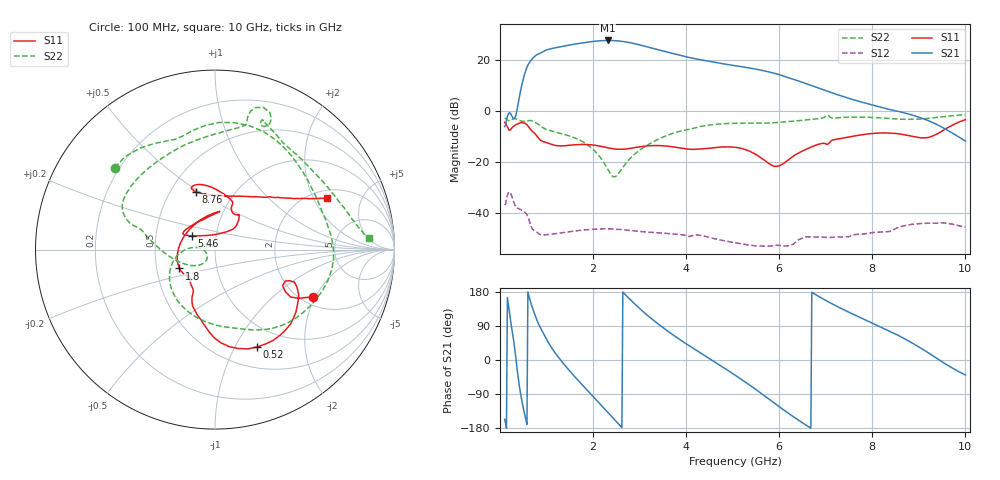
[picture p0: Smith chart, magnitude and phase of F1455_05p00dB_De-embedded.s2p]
! Integrated Device Technology
! Corporate Headquarters
! 6024 Silver Creek Valley Road
! San Jose, CA 95138  USA
! Phone:  1-408-284-8200
! Toll Free:  1-800-223-1366
! Webpage:  http://www.idt.com/
! Timing and RF Division
! 515 Groton Road, Suite 102
! Westford, MA 01886-6024
! Device:  F1455
! Description: 6-bit 0.5 dB Transmit Variable Gain Amplifier
! Frequency:  1400.0 -  2300.00 MHz
! Package:  6x6 mm Thin QFN Plastic Package: 28 pin
! State:  10
! Atten State:  5.0 dB
! Voltage:  +5.00 Volts
! Current:  216.802 mA
! Data:  The device was measured on a the F1455 evaluation board which has
!  individual transmission lines to the RF pins.  Data was collected
!  using a calibrated network analyzer.  The evaluation board was
!  de-embedded using a TRL calibration technique.
!  The reference plane is the edge of the package pin.
!  Pin  1 = CSb
!  Pin  2 = DATA
!  Pin  3 = CLK
!  Pin  4 = RSET
!  Pin  5 = GND
!  Pin  6 = RFIN  = Port 1
!  Pin  7 = GND
!  Pin  8 = NC
!  Pin  9 = NC
!  Pin 10 = NC
!  Pin 11 = NC
!  Pin 12 = NC
!  Pin 13 = NC
!  Pin 14 = /STBY
!  Pin 15 = GND
!  Pin 16 = RFOUT  = Port 2
!  Pin 17 = GND
!  Pin 18 = NC
!  Pin 19 = NC
!  Pin 20 = NC
!  Pin 21 = GND
!  Pin 22 = NC
!  Pin 23 = GND
!  Pin 24 = NC
!  Pin 25 = NC
!  Pin 26 = NC
!  Pin 27 = GND
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# GHz S dB R 50
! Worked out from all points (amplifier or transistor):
!   496 points, 100 MHz to 10 GHz, reference 50 ohm
!   highest |S21| = 27.8 dB at 2.32 GHz (marker M1)
!   |S21| within 3 dB of that: 1.159 GHz to 3.266 GHz (2.107 GHz wide, 95.3 % of centre)
!   unconditionally stable (mu >= 1): start of sweep to end of sweep
!   at 1.74 GHz: K = 4.40, MAG = 27.3 dB, |S12| = -46.7 dB
!   at 5.06 GHz: K = 15.28, MAG = 19.9 dB, |S12| = -51.6 dB
!   at 10 GHz: K = 48.04, MAG = -3.0 dB, |S12| = -45.4 dB
!   S11 on the Smith chart (normalised r, x): 100 MHz: 2.29, -1.92; 520 MHz: 0.74, -1.23; 1.8 GHz: 0.66, -0.15; 5.46 GHz: 0.76, +0.12; 8.76 GHz: 0.67, +0.48; 10 GHz: 2.34, +2.55
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0.1  -4.33 -25.8  -5.96 -156.3  -36.73 41.8  -2.84 140.8
0.4  -4.74 -40.8  3.90 -54.6  -38.14 -114.1  -3.43 50.4
0.52  -4.57 -66.8  14.01 -137.6  -39.37 -153.8  -3.96 23.7
0.7  -7.94 -101.0  20.70 137.1  -46.22 153.2  -3.86 -20.9
0.82  -10.32 -114.9  22.43 97.6  -47.77 138.1  -5.04 -49.5
0.96  -12.07 -119.7  23.76 64.1  -48.50 123.3  -6.79 -73.8
1.14  -13.14 -129.2  24.73 26.9  -48.09 100.0  -7.88 -98.1
1.34  -13.51 -134.1  25.48 -5.8  -47.59 77.9  -8.84 -121.6
1.76  -12.97 -150.0  26.81 -64.6  -46.63 42.0  -11.73 -159.9
1.8  -12.98 -152.1  26.92 -69.8  -46.53 38.9  -12.15 -163.1
2.06  -13.36 -169.1  27.53 -104.1  -46.18 20.8  -15.97 179.1
2.32  -14.33 165.4  27.80 -138.7  -46.10 3.7  -22.86 177.5
2.7  -14.79 118.5  27.25 171.7  -46.55 -18.2  -20.47 -129.6
3.02  -13.84 91.9  25.99 133.7  -47.14 -32.8  -14.98 -151.9
3.4  -13.41 83.0  24.16 95.0  -47.66 -47.1  -10.96 -176.7
4.1  -14.91 110.6  20.99 34.9  -48.88 -69.5  -6.90 164.0
5.06  -14.12 154.0  17.89 -40.6  -51.56 -104.2  -4.67 148.4
5.46  -16.49 149.2  16.69 -74.4  -52.73 -109.8  -4.65 133.9
6.7  -13.90 50.6  10.06 178.7  -49.23 -141.4  -3.13 78.3
8.36  -8.53 109.4  0.76 76.4  -47.15 166.5  -2.78 62.1
8.76  -9.43 108.2  -0.93 51.4  -44.62 152.7  -3.14 47.7
10  -3.28 24.9  -11.66 -39.5  -45.41 79.6  -1.29 4.5
